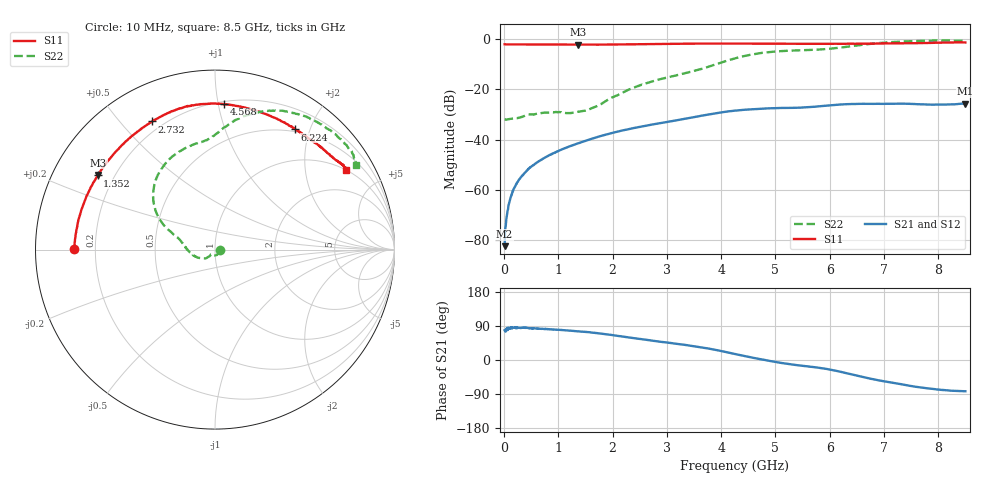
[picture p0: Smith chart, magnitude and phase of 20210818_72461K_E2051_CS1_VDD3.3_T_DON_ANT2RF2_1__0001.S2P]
!Agilent Technologies,E5071C,MY46417908,A.11.23
!Date: Wed Aug 18 14:27:10 2021
!Data & Calibration Information:
!Freq	S11:SOLT2(ON)	S21:SOLT2(ON)	S12:SOLT2(ON)	S22:SOLT2(ON)
!PortZ  Port1:50+j0  Port2:50+j0
!Above PortZ is port z conversion or system Z0 setting when saving the data.
!When reading, reference impedance value at option line is always used.
# Hz S dB R 50
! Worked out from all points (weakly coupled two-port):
!   1601 points, 10 MHz to 8.5 GHz, reference 50 ohm
!   highest |S21| = -25.64 dB at 8.495 GHz (marker M1); lowest = -82.3 dB at 10 MHz (marker M2)
!   lowest |S11| = -2.2 dB at 1.368 GHz (marker M3), VSWR 7.77, Z = 6.97 + j14.4 ohm
!   |S11| at or under -10 dB: nowhere
!   |S22| runs from -32.0 to -0.6 dB; largest |S21 - S12| = 0.00026
!   S11 on the Smith chart (normalised r, x): 10 MHz: 0.12, +0.00; 1.352 GHz: 0.14, +0.28; 2.732 GHz: 0.16, +0.61; 4.568 GHz: 0.22, +1.04; 6.224 GHz: 0.47, +1.78; 8.5 GHz: 0.99, +3.30
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1e7  -2.09 179.7  -82.29 78.5  -84.60 81.3  -31.80 -2.7
7.3675e7  -2.12 178.3  -67.63 83.7  -67.30 85.2  -31.92 -12.3
1.214312e8  -2.12 177.2  -62.88 86.3  -62.97 84.9  -31.66 -18.8
2.01025e8  -2.15 175.4  -58.67 84.9  -58.66 85.2  -31.47 -29.8
3.230688e8  -2.16 172.5  -54.59 85.1  -54.49 84.8  -30.98 -50.6
4.822562e8  -2.17 168.9  -51.06 83.7  -51.01 83.4  -29.97 -71.9
7.210375e8  -2.20 163.1  -47.51 82.1  -47.49 82.2  -29.29 -97.2
1.352481e9  -2.23 147.7  -41.49 75.7  -41.53 75.8  -28.91 -131.1
1.3684e9  -2.25 147.4  -41.42 75.8  -41.41 75.6  -28.88 -131.1
1.426769e9  -2.23 145.8  -40.98 74.9  -40.97 74.9  -28.72 -130.1
2.732106e9  -1.99 116.1  -33.96 51.0  -33.94 51.0  -16.82 -175.5
2.843538e9  -1.96 114.2  -33.53 48.9  -33.54 48.9  -16.11 179.1
3.803969e9  -1.80 99.2  -29.84 29.1  -29.83 29.2  -10.72 156.3
4.255e9  -1.79 91.8  -28.45 15.8  -28.46 15.8  -7.69 144.8
4.568069e9  -1.81 86.3  -27.91 6.4  -27.90 6.4  -6.12 133.2
5.098694e9  -1.86 75.9  -27.38 -7.5  -27.38 -7.5  -4.80 112.5
5.671769e9  -1.87 65.0  -26.97 -18.0  -26.97 -17.9  -4.31 95.5
6.223619e9  -1.88 56.2  -25.98 -31.9  -25.98 -32.0  -3.32 85.7
7.088538e9  -1.73 45.3  -25.73 -58.3  -25.76 -58.4  -1.28 63.3
7.916312e9  -1.49 36.0  -26.05 -76.6  -26.03 -76.7  -0.59 40.9
8.494694e9  -1.34 31.2  -25.64 -82.6  -25.64 -82.7  -0.76 31.2
8.5e9  -1.35 31.3  -25.64 -82.5  -25.66 -82.7  -0.77 31.1
